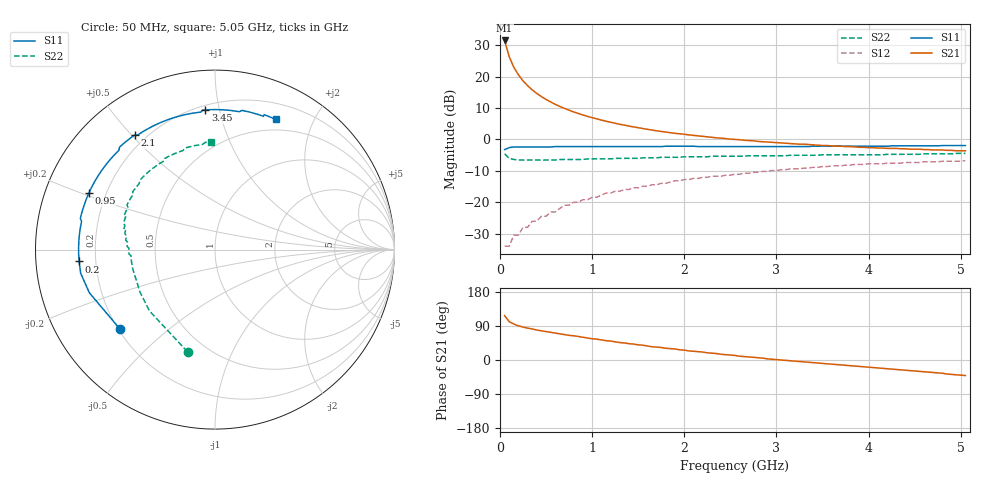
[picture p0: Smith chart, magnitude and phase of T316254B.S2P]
!AT-31625
!S-PARAMETERS at Vce=3.6 V  Ic=100 mA.  LAST UPDATED 08-05-96
# ghz s ma r 50
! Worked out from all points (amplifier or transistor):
!   101 points, 50 MHz to 5.05 GHz, reference 50 ohm
!   highest |S21| = 31.5 dB at 50 MHz (marker M1)
!   |S21| within 3 dB of that: start of sweep to 78.95 MHz
!   unconditionally stable (mu >= 1): 398.4 MHz to 405.9 MHz; 463.9 MHz to 1.748 GHz
!   at 850 MHz: K = 1.04, MAG = 12.9 dB, |S12| = -20.0 dB
!   at 2.55 GHz: K = 0.97, MSG = 5.5 dB, |S12| = -11.1 dB
!   at 5.05 GHz: K = 0.94, MSG = 1.6 dB, |S12| = -6.7 dB
!   S11 on the Smith chart (normalised r, x): 50 MHz: 0.21, -0.35; 200 MHz: 0.14, -0.04; 950 MHz: 0.14, +0.21; 2.1 GHz: 0.16, +0.51; 3.45 GHz: 0.23, +0.91; 5.05 GHz: 0.37, +1.50
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0.05  0.69 -140.0  37.64 117.0  0.02 42.0  0.59 -105.0
0.1  0.74 -161.0  20.73 101.0  0.02 41.0  0.5 -137.0
0.15  0.76 -170.0  14.09 95.0  0.03 46.0  0.48 -151.0
0.2  0.76 -175.0  10.65 90.0  0.03 50.0  0.47 -159.0
0.25  0.76 -178.0  8.56 87.0  0.04 54.0  0.47 -163.0
0.3  0.76 179.0  7.16 84.0  0.04 57.0  0.47 -166.0
0.35  0.76 176.0  6.15 82.0  0.05 59.0  0.47 -169.0
0.4  0.76 174.0  5.39 79.0  0.05 60.0  0.47 -171.0
0.45  0.76 172.0  4.8 77.0  0.06 61.0  0.47 -173.0
0.55  0.76 168.0  3.95 73.0  0.07 62.0  0.47 -175.0
0.65  0.77 165.0  3.35 69.0  0.08 63.0  0.48 -177.0
0.75  0.77 162.0  2.92 65.0  0.09 63.0  0.48 -179.0
0.9  0.77 157.0  2.45 60.0  0.11 62.0  0.48 179.0
0.95  0.77 156.0  2.33 58.0  0.11 61.0  0.49 178.0
1.3  0.77 146.0  1.74 46.0  0.15 57.0  0.5 173.0
1.75  0.77 134.0  1.34 33.0  0.2 50.0  0.52 168.0
2.1  0.78 125.0  1.16 23.0  0.24 44.0  0.53 163.0
2.55  0.77 114.0  1 12.0  0.28 37.0  0.54 156.0
3.4  0.78 95.0  0.82 -7.0  0.36 21.0  0.56 140.0
3.45  0.78 94.0  0.81 -8.0  0.36 20.0  0.56 139.0
4.25  0.79 79.0  0.72 -24.0  0.42 3.0  0.58 117.0
5.05  0.8 65.0  0.66 -41.0  0.46 -14.0  0.6 92.0
